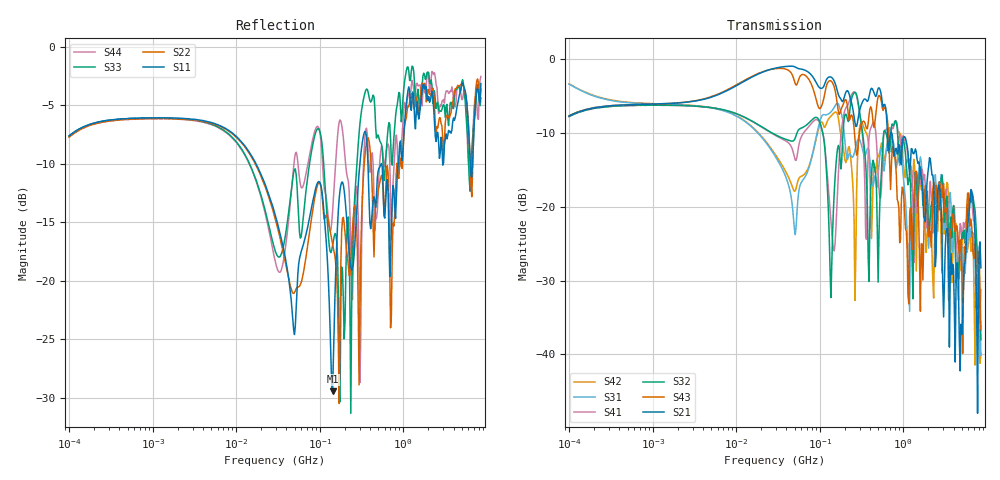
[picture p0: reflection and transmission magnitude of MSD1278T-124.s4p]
# MHz S MA R 50
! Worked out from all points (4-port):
!   498 points, 100 kHz to 8.5 GHz, reference 50 ohm
!   strongest paths, dB at 100 kHz, 1.698 MHz, 29.49 MHz, 500.7 MHz, 8.5 GHz:
!     S21: -7.7, -6.0, -1.2, -3.9, -28.3
!     S43: -7.7, -6.0, -1.2, -5.1, -36.7
!     S32: -7.7, -6.2, -10.2, -30.2, -38.0
!     S41: -7.7, -6.2, -10.3, -15.6, -31.2
!     S31: -3.4, -6.1, -13.2, -15.7, -40.2
!     S42: -3.3, -6.1, -12.9, -13.2, -39.9
!   lowest |S11| = -29.4 dB at 142.6 MHz (marker M1), VSWR 1.07, Z = 53.5 - j0.45 ohm
!   |S11| at or under -10 dB: 17.23 MHz to 302.6 MHz (285.4 MHz wide, 178 % of centre); 377.7 MHz to 547.4 MHz (169.7 MHz wide, 36.7 % of centre); 549 MHz to 872 MHz (323 MHz wide, 45.5 % of centre)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
0.1  0.4157 31.6  0.4135 32.7  0.6793 -19.4  0.4099 -148.1
     0.4135 32.7  0.4107 31.8  0.41 -148.1  0.6826 -19.2
     0.6793 -19.4  0.41 -148.1  0.4153 31.7  0.4142 32.6
     0.4099 -148.1  0.6826 -19.2  0.4142 32.6  0.4109 32.0
142.5721  0.03371 -7.2  0.7438 -40.8  0.4544 37.0  0.05797 -99.9
          0.7438 -40.8  0.1436 -69.4  0.06586 66.8  0.4241 42.3
          0.4544 37.0  0.06586 66.8  0.1412 -32.2  0.6936 -49.3
          0.05797 -99.9  0.4241 42.3  0.6936 -49.3  0.1973 9.9
258.1735  0.1288 159.2  0.4061 -61.9  0.2288 -28.2  0.604 -4.7
          0.4061 -61.9  0.2038 58.0  0.5933 -22.6  0.07944 -68.9
          0.2288 -28.2  0.5933 -22.6  0.2042 81.7  0.3395 -78.8
          0.604 -4.7  0.07944 -68.9  0.3395 -78.8  0.1641 -2.3
1088.348  0.5681 -82.2  0.2771 -150.8  0.08839 -178.7  0.2632 -149.8
          0.2771 -150.8  0.4967 -80.3  0.1909 -165.4  0.1984 -130.8
          0.08839 -178.7  0.1909 -165.4  0.7897 -99.6  0.06807 179.7
          0.2632 -149.8  0.1984 -130.8  0.06807 179.7  0.5415 -91.1
2260.241  0.6151 160.8  0.1642 63.6  0.06644 134.0  0.06811 111.2
          0.1642 63.6  0.6655 167.5  0.1011 129.0  0.03154 94.2
          0.06644 134.0  0.1011 129.0  0.5721 154.2  0.1308 172.5
          0.06811 111.2  0.03154 94.2  0.1308 172.5  0.7772 166.8
3488.216  0.4386 26.5  0.04428 69.2  0.08576 18.4  0.0676 -20.3
          0.04428 69.2  0.4976 15.3  0.06593 -18.1  0.1084 -33.5
          0.08576 18.4  0.06593 -18.1  0.4604 10.4  0.02326 -173.6
          0.0676 -20.3  0.1084 -33.5  0.02326 -173.6  0.6316 9.4
8500  0.6956 -31.6  0.03858 -126.9  0.009803 -116.0  0.02744 -80.6
      0.03858 -126.9  0.6579 -40.6  0.01255 61.4  0.01012 -103.9
      0.009803 -116.0  0.01255 61.4  0.604 -37.4  0.01467 -123.5
      0.02744 -80.6  0.01012 -103.9  0.01467 -123.5  0.7458 -40.5
